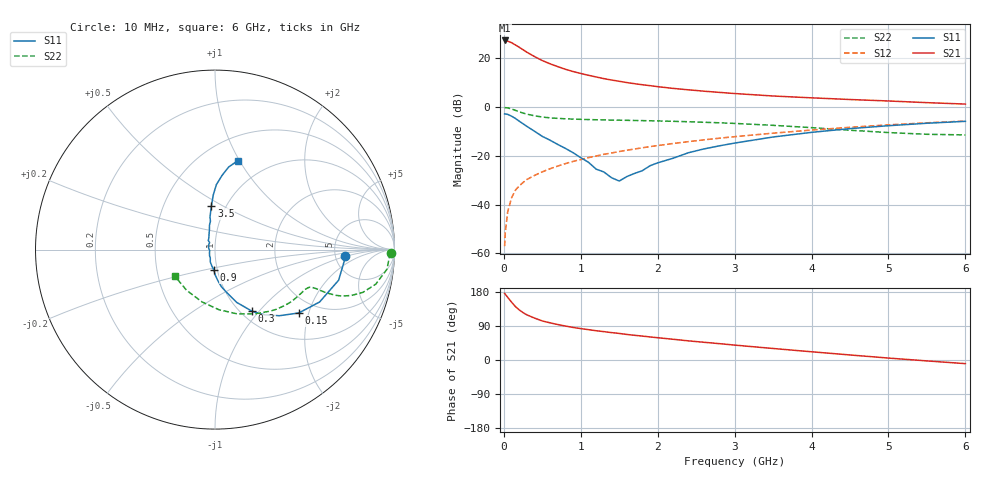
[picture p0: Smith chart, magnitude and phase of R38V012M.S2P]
! SIEMENS Small Signal Semiconductors
! BFR181
! Si NPN RF Bipolar Junction Transistor in SOT23
! VCE = 8 V  IC = 12 mA
! Common Emitter S-Parameters:  May  1996
# GHz  S  MA  R  50
!  f  S11  S21  S12  S22
! GHz  MAG  ANG  MAG  ANG  MAG  ANG  MAG  ANG
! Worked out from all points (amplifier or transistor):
!   36 points, 10 MHz to 6 GHz, reference 50 ohm
!   highest |S21| = 27.3 dB at 10 MHz (marker M1)
!   |S21| within 3 dB of that: start of sweep to 210.6 MHz
!   unconditionally stable (mu >= 1): 808.6 MHz to 2.735 GHz
!   at 250 MHz: K = 0.63, MSG = 27.2 dB, |S12| = -30.9 dB
!   at 1.4 GHz: K = 1.05, MAG = 13.6 dB, |S12| = -18.8 dB
!   at 6 GHz: K = 0.86, MSG = 3.5 dB, |S12| = -5.7 dB
!   S11 on the Smith chart (normalised r, x): 10 MHz: 6.14, -0.92; 150 MHz: 1.61, -1.73; 300 MHz: 1.12, -0.92; 900 MHz: 0.96, -0.23; 3.5 GHz: 0.86, +0.44; 6 GHz: 0.73, +0.98
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0.01  0.7253 -2.8  23.31 175.8  0.0014 89.0  0.981 -1.1
0.02  0.7222 -5.4  22.78 173.3  0.0028 90.5  0.9721 -2.5
0.05  0.7096 -13.9  22.56 165.5  0.0071 82.9  0.9645 -6.5
0.1  0.6518 -26.6  21 152.7  0.0137 79.3  0.9166 -12.1
0.15  0.5852 -37.1  18.86 141.1  0.0197 73.9  0.8583 -16.1
0.2  0.5139 -45.8  16.92 132.2  0.0242 72.3  0.8016 -18.6
0.25  0.455 -52.9  15.02 124.9  0.0284 69.6  0.7531 -20.1
0.3  0.4017 -58.9  13.34 119.1  0.0327 70.1  0.7161 -20.8
0.4  0.3185 -67.6  10.87 110.5  0.0397 69.4  0.6624 -21.2
0.5  0.2506 -74.4  9.014 103.1  0.0469 70.1  0.625 -21.2
0.6  0.2094 -80.3  7.74 98.1  0.0543 70.6  0.602 -21.1
0.7  0.1715 -85.0  6.778 93.6  0.0616 70.8  0.5869 -21.2
0.9  0.1159 -92.9  5.371 85.9  0.0768 70.5  0.5671 -21.7
1.1  0.0738 -110.8  4.496 80.1  0.0917 70.5  0.5547 -23.0
1.3  0.0467 -130.1  3.84 74.9  0.1074 69.7  0.5456 -24.6
1.5  0.0304 -167.5  3.388 70.1  0.1226 69.2  0.539 -26.6
1.8  0.0495 127.0  2.878 63.1  0.1461 67.5  0.5278 -29.9
2.2  0.0892 111.9  2.419 54.7  0.179 65.0  0.5111 -35.2
3.5  0.2435 94.8  1.69 30.4  0.2916 54.1  0.4225 -58.0
4.5  0.362 88.8  1.431 13.3  0.3852 43.3  0.3353 -86.4
5.5  0.4667 80.6  1.234 -2.4  0.4757 30.9  0.2766 -124.9
6  0.5104 75.7  1.153 -9.6  0.517 24.1  0.2686 -146.9
